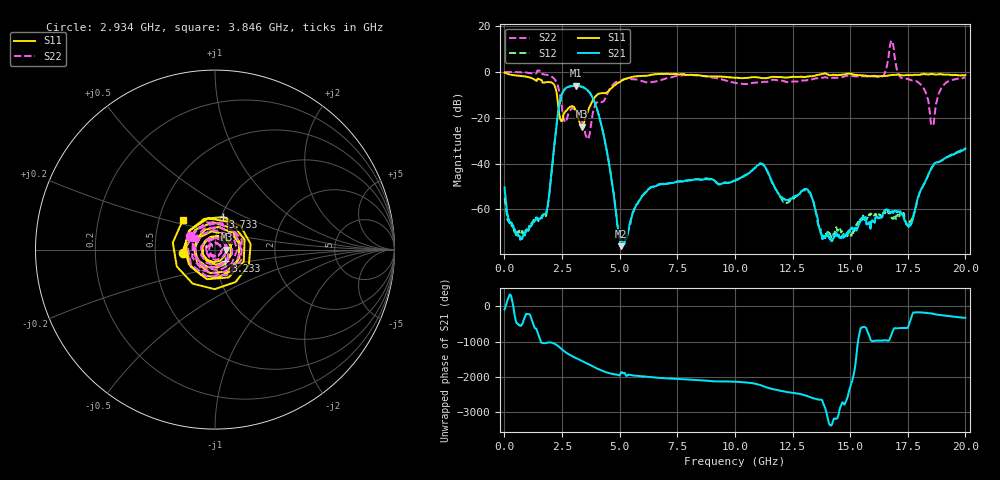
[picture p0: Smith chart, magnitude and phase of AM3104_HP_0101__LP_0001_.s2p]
!Created with skrf (http://scikit-rf.org).
# Hz S RI R 50.0
!freq ReS11 ImS11 ReS21 ImS21 ReS12 ImS12 ReS22 ImS22
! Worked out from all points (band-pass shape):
!   1601 points, 10 MHz to 20 GHz, reference 50 ohm
!   highest |S21| = -6.02 dB at 3.108 GHz (marker M1); lowest = -76.0 dB at 5.07 GHz (marker M2)
!   |S21| within 3 dB of the highest: 2.526 GHz to 3.701 GHz (1.175 GHz wide, 37.7 % of centre)
!   lowest |S11| = -24.0 dB at 3.346 GHz (marker M3), VSWR 1.14, Z = 56.8 - j0.119 ohm
!   |S11| at or under -10 dB: 2.281 GHz to 4.027 GHz (1.746 GHz wide, 55.4 % of centre)
!   |S22| runs from -29.3 to 13.7 dB; largest |S21 - S12| = 0.027
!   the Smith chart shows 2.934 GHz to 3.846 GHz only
!   S11 on the Smith chart (normalised r, x): 2.934 GHz: 0.70, -0.02; 3.233 GHz: 1.11, -0.15; 3.733 GHz: 1.02, +0.38; 3.846 GHz: 0.66, +0.23
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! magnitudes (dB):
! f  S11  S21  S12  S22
! 10 MHz  -0.3  -50.5  -54.9  -0.1
! 697.2 MHz  -1.8  -72.8  -69.7  -0.2
! 1.734 GHz  -4.6  -62.0  -62.5  -1.2
! 2.421 GHz  -20.4  -12.5  -12.6  -10.6
! 2.934 GHz  -15.0  -6.1  -6.2  -16.0
! 3.108 GHz  -17.0  -6.0  -6.0  -17.1
! 3.233 GHz  -21.2  -6.1  -6.2  -18.8
! 3.346 GHz  -24.0  -6.4  -6.5  -20.8
! 3.733 GHz  -14.6  -9.5  -9.5  -24.6
! 3.846 GHz  -12.3  -11.6  -11.6  -17.6
! 5.07 GHz  -4.0  -76.0  -73.8  -3.7
! 6.682 GHz  -0.9  -49.3  -49.1  -3.9
! 10.01 GHz  -2.6  -47.4  -47.5  -4.8
! 11.15 GHz  -2.8  -40.0  -40.2  -4.5
! 12.15 GHz  -2.5  -55.6  -56.8  -4.2
! 13.34 GHz  -2.0  -54.8  -54.8  -3.3
! 14.19 GHz  -1.4  -73.8  -71.9  -2.7
! 16.68 GHz  -1.6  -60.7  -61.7  7.2
! 17.6 GHz  -1.5  -67.1  -65.1  -3.5
! 18.56 GHz  -0.9  -41.3  -41.4  -23.3
! 19.01 GHz  -1.2  -38.3  -38.5  -6.3
! 20 GHz  -1.4  -33.6  -33.4  -2.5
